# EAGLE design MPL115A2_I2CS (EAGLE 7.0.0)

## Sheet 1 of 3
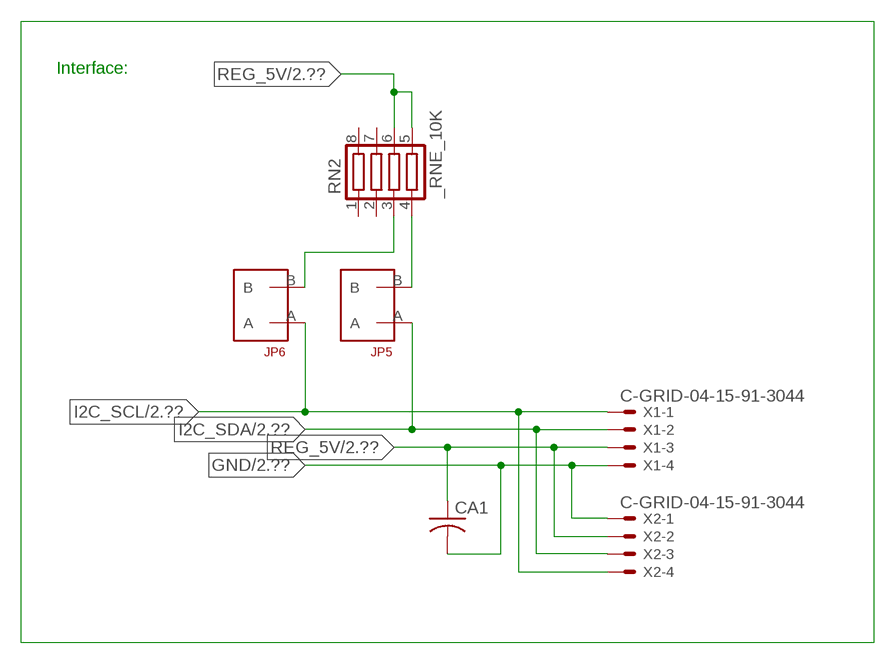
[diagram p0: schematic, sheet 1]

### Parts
CA1  CC1206KRX7R9BB104  [.1UF]
JP5  JUMPER_1X2_2MM  [JUMPER_1X2_2MM]
JP6  JUMPER_1X2_2MM  [JUMPER_1X2_2MM]
RN2  _RNE_10K  [RNE]
X1  C-GRID-04-15-91-3044  [15-91-04]
X2  C-GRID-04-15-91-3044  [15-91-04]

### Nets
GND: CA1.2 X1.4 X2.1 ; also sheet 2,3
I2C_SCL: JP6.A X1.1 X2.4 ; also sheet 2
I2C_SDA: JP5.A X1.2 X2.3 ; also sheet 2
N$1: JP6.B RN2.3
N$2: JP5.B RN2.4
REG_5V: CA1.1 RN2.5 RN2.6 X1.3 X2.2 ; also sheet 2,3
Unconnected: RN2.1 RN2.2 RN2.7 RN2.8

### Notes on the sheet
- Interface:

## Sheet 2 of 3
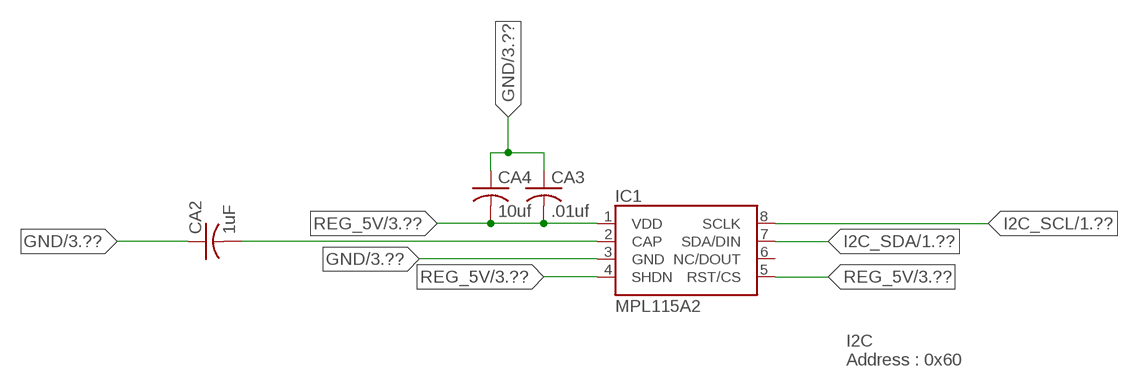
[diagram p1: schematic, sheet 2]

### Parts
CA2  1uF  CC0603JRNPO8BN1020603  [CC0603JRNPO8BN102]
CA3  .01uf  CC1206KRX7R9BB104C1206K  [CC1206KRX7R9BB104]
CA4  10uf  CC1206KRX7R9BB104C1206K  [CC1206KRX7R9BB104]
IC1  MPL115A2  MPL115A  [LGA8]

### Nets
GND: CA2.1 CA3.1 CA4.1 IC1.3(GND) ; also sheet 1,3
I2C_SCL: IC1.8(SCLK) ; also sheet 1
I2C_SDA: IC1.7(SDA/DIN) ; also sheet 1
N$14: CA2.2 IC1.2(CAP)
REG_5V: CA3.2 CA4.2 IC1.1(VDD) IC1.4(SHDN) IC1.5(RST/CS) ; also sheet 1,3
Unconnected: IC1.6(NC/DOUT)

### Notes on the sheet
- I2C 
  Address : 0x60

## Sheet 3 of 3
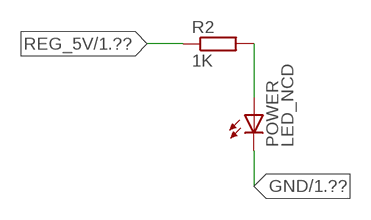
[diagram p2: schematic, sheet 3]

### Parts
POWER  LED_NCD  [CHIPLED_0603]
R2  1K  RESISTOR_SMT-0402  [R402]

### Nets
GND: POWER.C ; also sheet 1,2
N$3: POWER.A R2.2
REG_5V: R2.1 ; also sheet 1,2

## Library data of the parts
CA1 CA3 CA4 = NCD_ULTIMATE_LIBRARY:CC1206KRX7R9BB104: Capacitor CA .1uF 50V SMT C1206K CC1206KRX7R9BB104
CA2 = NCD_ULTIMATE_LIBRARY:CC0603JRNPO8BN102: Capacitor CE 1uF SMT CC0603JRNPO8BN102 0603
IC1 = NCD_ULTIMATE_ROHIT:MPL115A: MPL115A1 (SPI) and MPL115A2 (I2C) Miniature Digital Barometer 5.0x3.0x1.2mm LGA Package
JP5 JP6 = NCD_ULTIMATE_CONNECTORS:JUMPER_1X2_2MM
POWER = NCD_ULTIMATE_LIBRARY:LED_NCD: LED Digikey 754-1132-2-ND/APT2012SRCPRV
R2 = NCD_ULTIMATE_LIBRARY:RESISTOR_SMT: NCD Resistor
RN2 = NCD_ULTIMATE_LIBRARY:_RNE_10K: Resistor Array RNE SMT 10K x 4 Single Resistor Source: http://www.ctscorp.com/components/Datasheets/CTSChipArrayDs.pdf Digikey 742C083103JPTR-ND/742C083103JP; OC_FARNELL: unknown; OC_NEWARK: unknown
X1 X2 = NCD_ULTIMATE_CONNECTORS:C-GRID-04: CONNECTOR 4-Pos I2C wire to board 2.54 mm (0.100") pitch header Digikey WM1342-ND/0015912045; OC_FARNELL: unknown; OC_NEWARK: unknown

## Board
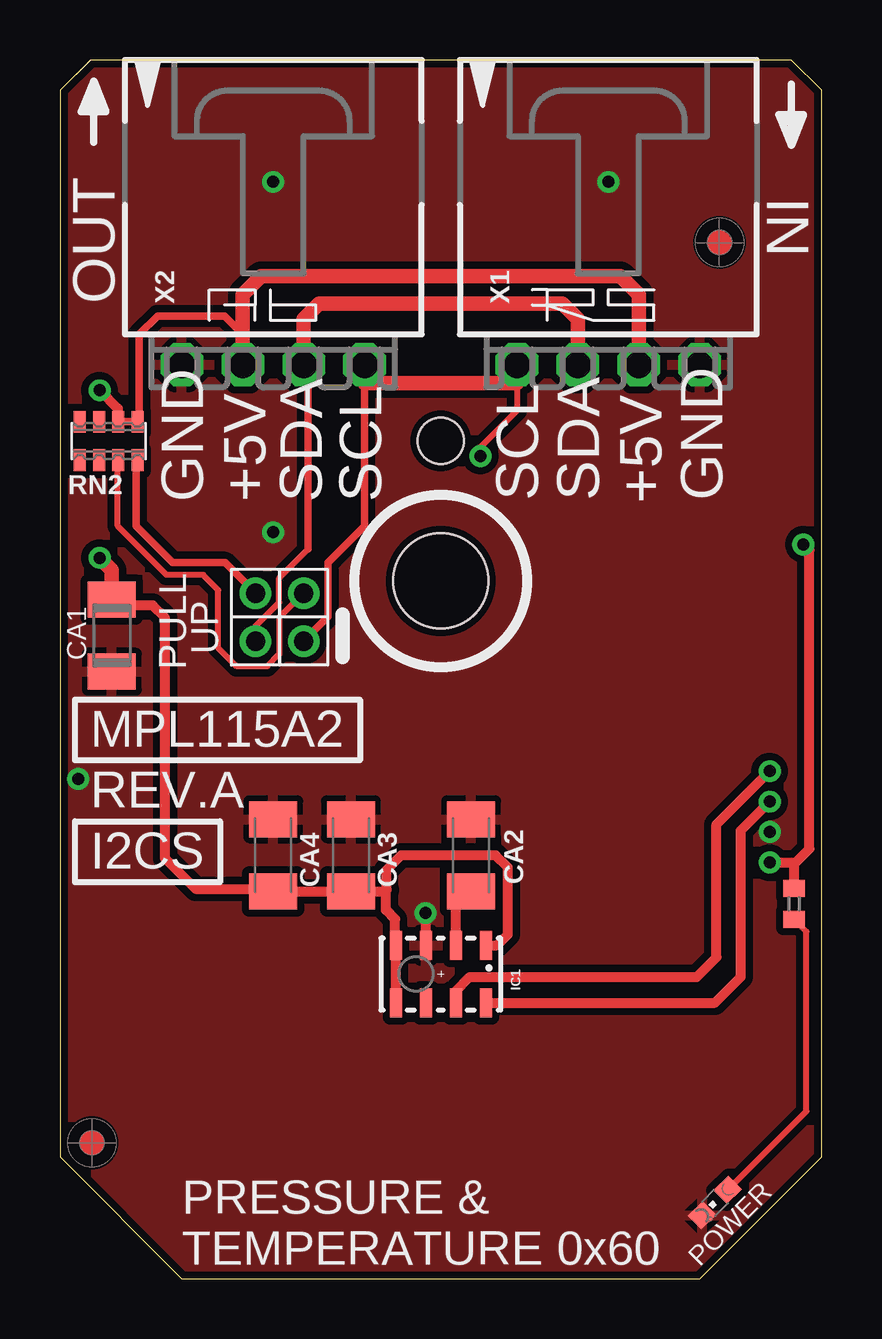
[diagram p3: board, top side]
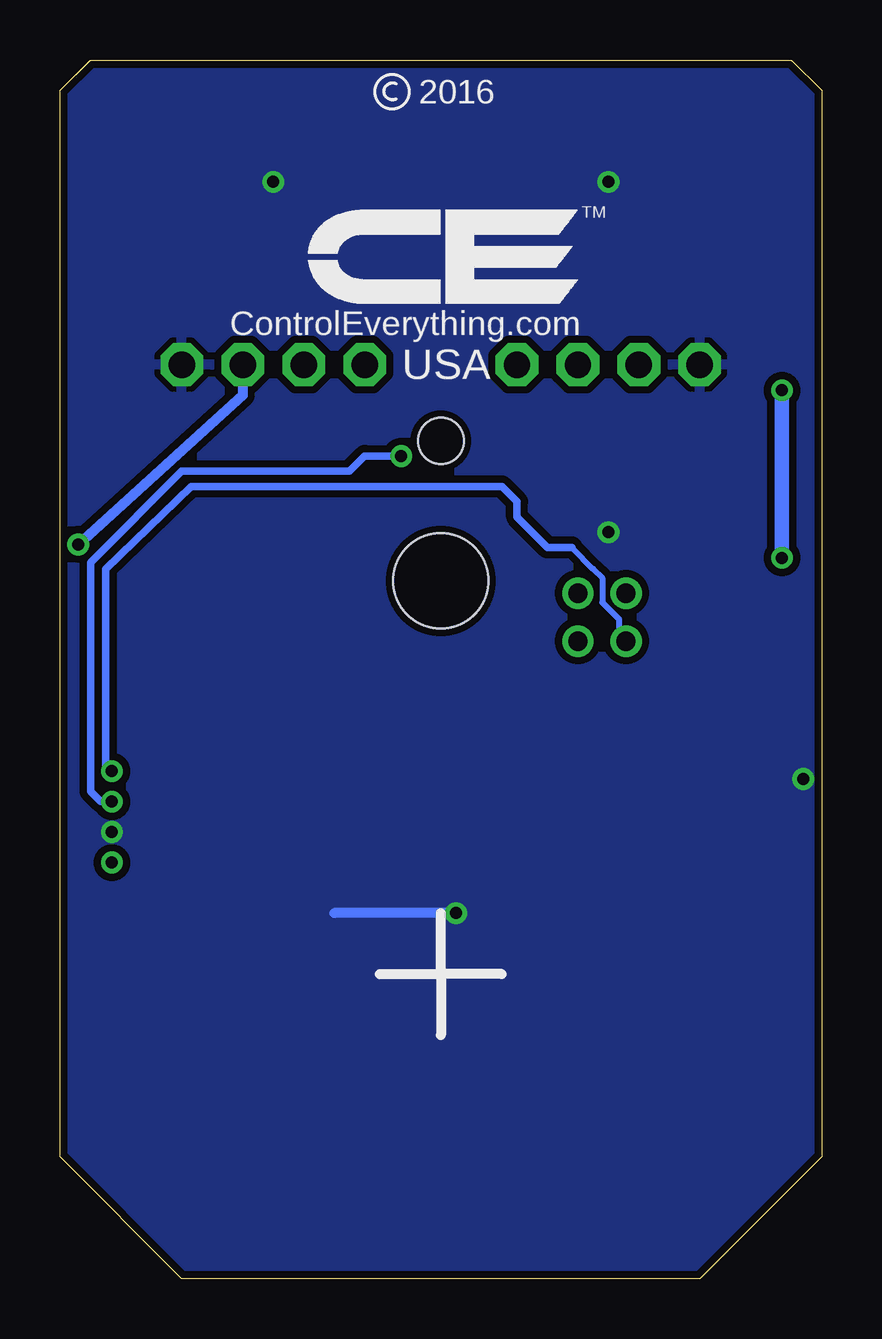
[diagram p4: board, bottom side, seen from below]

Size 31.75 x 50.8 mm. Coordinates in mm from the lower left corner, seen from the top.
Outline: 40 segments
Copper layers (1*16): Top 0.035mm / dielectric 1.5mm / Bottom 0.035mm
Design rules "default": minimum track width 5mil, minimum drill 24mil, track to track 5mil, track to pad 5mil, pad to pad 5mil, via to via 5mil, smd to smd 5mil, copper to edge 10mil, drill to drill 8mil, minimum pad ring 10mil, minimum via ring 8mil, stop-mask expansion 2mil, vias tented up to drill 0mil, thermal gap 10mil
Holes 3.96 mm at 15.88,29.08
Holes 1.91 mm at 15.88,34.92

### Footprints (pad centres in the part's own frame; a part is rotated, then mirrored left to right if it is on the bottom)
.1UF = smd 1.5 x 2: 1 -1.5,0; 2 1.5,0
CC0603JRNPO8BN102 = smd 1.5 x 2: 1 -1.5,0; 2 1.5,0
CC1206KRX7R9BB104 = smd 1.5 x 2: 1 -1.5,0; 2 1.5,0
LGA8 = smd 1.2 x 0.5: 1 -1.2,1.875; 2 -1.2,0.625; 3 -1.2,-0.625; 4 -1.2,-1.875; 5 1.2,-1.875; 6 1.2,-0.625; 7 1.2,0.625; 8 1.2,1.875
JUMPER_1X2_2MM = drill 0.8: A 0,2; B 0,0
CHIPLED_0603 = smd 0.8 x 0.876: A 0,-0.75; C 0,0.75
R402 = smd 0.7 x 0.9: 1 -0.65,0; 2 0.65,0
RNE = smd 0.5 x 0.9: 1 -1.2,-0.8; 2 -0.4,-0.8; 3 0.4,-0.8; 4 1.2,-0.8; 5 1.2,0.8; 6 0.4,0.8; 7 -0.4,0.8; 8 -1.2,0.8
15-91-04 = drill 1.1 pad 1.778 octagon: 1 -3.81,-7.62; 2 -1.27,-7.62; 3 1.27,-7.62; 4 3.81,-7.62

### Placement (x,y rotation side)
CA1  2.16,26.81 270 top
CA2  17.15,17.65 270 top
CA3  12.13,17.65 270 top
CA4  8.89,17.65 270 top
IC1  15.88,12.7 270 top
JP5  8.15,28.58 180 top
JP6  10.16,28.58 180 top
POWER  27.3,3.18 135 top
R2  30.61,15.62 270 top
RN2  2.03,34.92 0 top
U$5  [VISION_REF10]  1.33,5.66 90 top
U$28  [VISION_REF10]  27.5,43.19 90 top
X1  22.86,45.72 0 top
X2  8.89,45.72 0 top

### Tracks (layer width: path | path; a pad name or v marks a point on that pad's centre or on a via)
GND  (via drill 0.5)
  Top 0.406: IC1.3 15.25,14.6 v15.24,15.24
  Bottom 0.406: v15.24,15.24 20.32,15.24
  other vias: 8.89,45.72 22.86,45.72 29.59,18.62 0.76,20.83 8.89,31.12
  pour Bottom (isolate 0.305): 4.45,-0.63 -0.63,4.45 -0.63,50.17 0.64,51.44 31.12,51.44 32.38,50.17 32.38,4.45 27.3,-0.63
  pour Top (isolate 0.305): 3.81,-1.27 -1.27,3.81 -1.27,50.8 0,52.07 31.75,52.07 33.02,50.8 33.02,3.81 27.94,-1.27
I2C_SCL  (via drill 0.5)
  Top 0.254: X1.1 19.05,36.2 17.53,34.67 v17.53,34.29
  Top 0.305: JP6.A 11.18,27.61 11.18,29.85 12.7,31.37 X2.4
  Top 0.406: X2.4 12.7,37.34 | 19.05,37.34 X1.1 | 29.39,19.69 v29.59,19.89 28.38,18.68 28.38,12.57 27.31,11.5 IC1.8
  Top 0.61: 12.7,37.34 19.05,37.34
  Bottom 0.305: v29.59,19.89 30.05,19.89 30.48,20.32 30.48,29.85 26.67,33.66 19.69,33.66 19.05,34.29 v17.53,34.29
I2C_SDA  (via drill 0.5)
  Top 0.254: JP5.A 8.15,27.2 9.14,28.19 9.14,29.21 10.35,30.42
  Top 0.305: 10.35,30.42 10.35,38.54 X2.3
  Top 0.406: 29.39,20.96 v29.59,21.16 27.37,18.94 27.37,13.4 26.54,12.57 17.08,12.57 16.5,11.99 IC1.7
  Top 0.61: X2.3 10.16,40.01 10.8,40.64 20.96,40.64 21.59,40.01 X1.2
  Bottom 0.254: 10.41,30.48 9.52,29.59 9.14,29.21 9.14,28.19 8.45,27.5 8.45,26.87 JP5.A
  Bottom 0.305: 10.41,30.48 11.43,30.48 12.7,31.75 12.7,32.39 13.34,33.02 26.29,33.02 29.85,29.59 29.85,21.41 v29.59,21.16
N$1
  Top 0.254: JP6.B | JP6.B 9.14,27.56 9.14,26.04 8.64,25.53 7.37,25.53 6.6,26.29 6.6,28.7 5.97,29.34 4.45,29.34 2.41,31.37 2.41,34.11 RN2.3
N$2
  Top 0.305: JP5.B 6.88,29.85 4.7,29.85 3.18,31.37 3.18,34.07 RN2.4
N$3
  Top 0.254: POWER.A 31.12,6.99 31.12,14.46 R2.2
N$14
  Top 0.406: IC1.2 16.5,16.14 CA2.2
REG_5V  (via drill 0.5)
  Top 0.305: 7.62,39.37 7.49,39.37 | RN2.6 RN2.5 3.3,35.8 3.3,39.37 4.06,40.13 6.86,40.13 7.62,39.37 | X2.2 7.62,39.37
  Top 0.406: v29.59,17.35 30.48,17.35 | 30.48,17.35 30.67,17.35 31.24,17.92 31.24,30.35 v30.99,30.61 | v1.65,37.03 2.41,36.27 2.41,35.74 RN2.6 | IC1.5 IC1.4 13.97,13.93 13.97,14.99 13.59,15.37 13.59,16.09 13.52,16.15 | CA1.1 2.4,28.07 3.87,28.07 4.38,27.56 4.38,17.53 5.65,16.26 8.79,16.26 CA4.2 CA3.2 13.52,16.15 | IC1.1 18.22,13.9 18.67,14.35 18.67,17.15 18.16,17.65 14.22,17.65 13.59,17.02 13.59,16.22 | 13.52,16.15 13.59,16.22 | 13.59,16.22 13.63,16.22 | R2.1 30.61,17.22 30.48,17.35
  Top 0.61: X1.3 v24.13,38.23 24.13,41.02 23.37,41.78 8.38,41.78 7.62,41.02 X2.2 | CA1.1 2.16,29.54 v1.65,30.05
  Bottom 0.406: v24.13,38.23 24.16,38.08 24.13,37.47 24.13,36.83 v30.99,30.61
  Bottom 0.61: v1.65,30.05 v1.65,37.03

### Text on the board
tNames: IN | OUT | GND | +5V | SDA | SCL | SCL | SDA | +5V | GND | UP | PULL | MPL115A2 | REV.A | I2CS | PRESSURE & / TEMPERATURE 0x60
bNames: 2016 | TM | ControlEverything.com | USA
